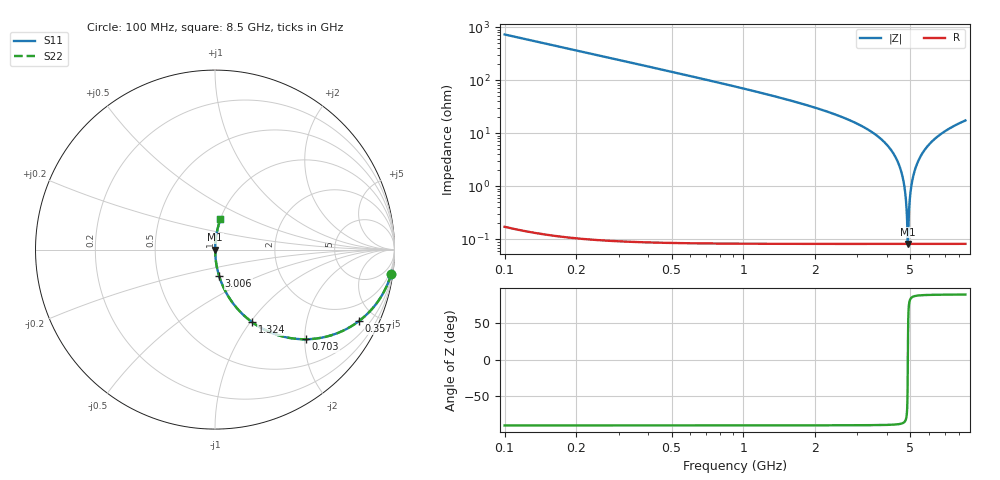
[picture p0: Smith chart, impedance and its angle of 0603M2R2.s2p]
! Created Wed Apr 18 15:27:35 2012
# hz S ma R 50
! 2 Port Network Data from SP1.SP block
! freq  magS11  angS11  magS21  angS21  magS12  angS12  magS22  angS22
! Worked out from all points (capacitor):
!   8401 points, 100 MHz to 8.5 GHz, reference 50 ohm
!   read as one part in series: C = 2.19 pF near 142 MHz
!   lowest |Z| = 82.1 mohm at 4.88 GHz (marker M1)
!   series resonance near 4.88 GHz, so ESL is about 490 pH
!   S11 on the Smith chart (normalised r, x): 100 MHz: 1, -15; 357 MHz: 1.00, -4.05; 703 MHz: 1.00, -2.02; 1.324 GHz: 1.00, -1.02; 3.006 GHz: 1.00, -0.30; 8.5 GHz: 1.00, +0.35
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1e8  0.9906 -7.8  0.1364 82.1  0.1364 82.1  0.9906 -7.8
2.21e8  0.9565 -16.9  0.2915 73.0  0.2915 73.0  0.9565 -16.9
3.57e8  0.8965 -26.3  0.4427 63.7  0.4427 63.7  0.8965 -26.3
7.03e8  0.7111 -44.6  0.7025 45.3  0.7025 45.3  0.7111 -44.6
1.324e9  0.453 -63.0  0.8908 26.9  0.8908 26.9  0.453 -63.0
1.5e9  0.4015 -66.2  0.9151 23.7  0.9151 23.7  0.4015 -66.2
2.9e9  0.1599 -80.5  0.9863 9.2  0.9863 9.2  0.1599 -80.5
3.006e9  0.1483 -81.2  0.9881 8.5  0.9881 8.5  0.1483 -81.2
3.787e9  0.07607 -85.0  0.9963 4.4  0.9963 4.4  0.07607 -85.0
4.3e9  0.03774 -86.6  0.9985 2.2  0.9985 2.2  0.03774 -86.6
4.534e9  0.02191 -86.6  0.9989 1.3  0.9989 1.3  0.02191 -86.6
4.694e9  0.01159 -85.3  0.9991 0.7  0.9991 0.7  0.01159 -85.3
4.784e9  0.005957 -81.7  0.9992 0.3  0.9992 0.3  0.005957 -81.7
4.854e9  0.001776 -62.4  0.9992 0.1  0.9992 0.1  0.001776 -62.4
4.88e9  0.0008205 1.1  0.9992 -0.0  0.9992 -0.0  0.0008205 1.1
4.905e9  0.001743 61.8  0.9992 -0.1  0.9992 -0.1  0.001743 61.8
4.987e9  0.006527 82.4  0.9992 -0.4  0.9992 -0.4  0.006527 82.4
5.115e9  0.01405 85.8  0.9991 -0.8  0.9991 -0.8  0.01405 85.8
5.347e9  0.02727 86.7  0.9988 -1.6  0.9988 -1.6  0.02727 86.7
5.7e9  0.04642 86.3  0.9981 -2.7  0.9981 -2.7  0.04642 86.3
7.1e9  0.1136 83.1  0.9927 -6.5  0.9927 -6.5  0.1136 83.1
8.5e9  0.1715 79.9  0.9844 -9.9  0.9844 -9.9  0.1715 79.9
